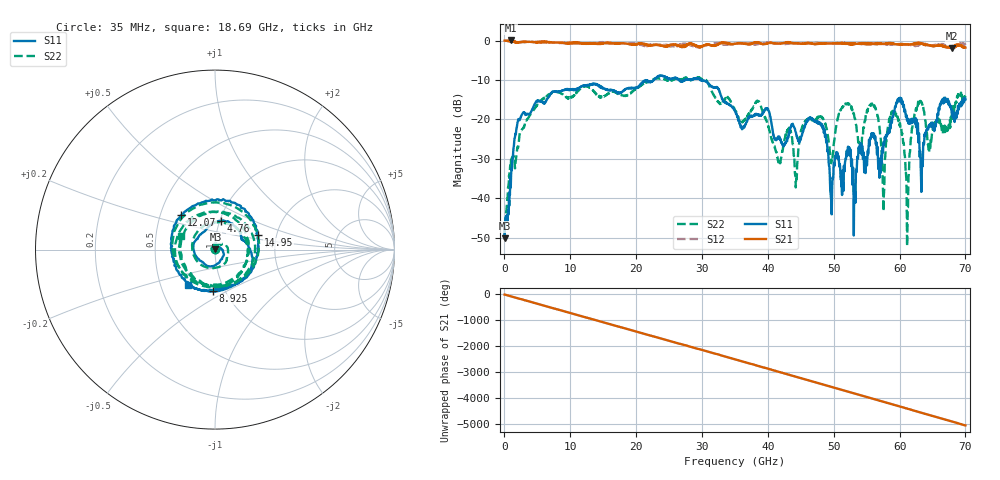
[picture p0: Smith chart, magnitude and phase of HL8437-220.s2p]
! 7/8/2021 2:28:10 PM
! H:\PROTOTYPE_DATA\DCBS_7-8-21\220NF_10V_CERAMIC_1.S2P
! CHANNEL.1
! TR.MEASUREMENT
! CORRECTED.DATA
# GHZ S RI R 50.0
! FREQ.GHZ  S11RE  S11IM  S21RE  S21IM  S12RE  S12IM  S22RE  S22IM
!; PortSelection: Port_12
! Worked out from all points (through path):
!   2000 points, 35 MHz to 70 GHz, reference 50 ohm
!   highest |S21| = 0.02 dB at 1.015 GHz (marker M1); lowest = -2.0 dB at 67.97 GHz (marker M2)
!   group delay of S21, straight-line fit = 201 ps
!   lowest |S11| = -50.2 dB at 35 MHz (marker M3), VSWR 1.01, Z = 50.3 + j0.143 ohm
!   |S11| at or under -10 dB: start of sweep to 22.68 GHz; 26.54 GHz to 27.43 GHz (892.7 MHz wide, 3.31 % of centre); 29.88 GHz to end of sweep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
!   |S22| runs from -52.2 to -9.3 dB; largest |S21 - S12| = 0.13
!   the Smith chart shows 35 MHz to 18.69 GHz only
!   S11 on the Smith chart (normalised r, x): 35 MHz: 1.01, +0.00; 4.76 GHz: 1.02, +0.34; 8.925 GHz: 0.88, -0.43; 12.07 GHz: 0.64, +0.27; 14.95 GHz: 1.60, +0.27; 18.69 GHz: 0.69, -0.29
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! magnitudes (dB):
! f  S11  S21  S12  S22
! 35 MHz  -50.2  0.0  0.0  -50.2
! 1.015 GHz  -34.3  0.0  -0.1  -30.3
! 4.76 GHz  -15.7  -0.4  -0.4  -16.8
! 8.925 GHz  -12.7  -0.6  -0.6  -13.8
! 11.72 GHz  -11.6  -0.7  -0.7  -11.9
! 12.07 GHz  -11.4  -0.8  -0.9  -11.6
! 14.95 GHz  -12.0  -0.7  -0.4  -14.2
! 18.69 GHz  -12.1  -0.8  -0.7  -13.8
! 23.38 GHz  -9.0  -1.1  -1.0  -9.6
! 35.03 GHz  -17.9  -0.8  -0.8  -17.7
! 44.27 GHz  -23.4  -0.7  -0.7  -36.1
! 46.69 GHz  -20.0  -0.8  -0.7  -20.0
! 49.63 GHz  -41.0  -0.7  -0.7  -31.1
! 55.86 GHz  -24.4  -0.8  -0.9  -16.4
! 57.58 GHz  -25.7  -0.8  -0.9  -43.4
! 58.34 GHz  -22.7  -0.6  -1.1  -21.0
! 59.99 GHz  -15.4  -1.0  -1.0  -21.6
! 61.15 GHz  -20.3  -1.0  -1.1  -52.2
! 62.86 GHz  -25.6  -0.9  -0.8  -15.8
! 64.54 GHz  -21.9  -1.3  -1.3  -26.8
! 67.97 GHz  -18.3  -2.0  -1.7  -17.5
! 70 GHz  -15.0  -1.8  -1.1  -14.0
